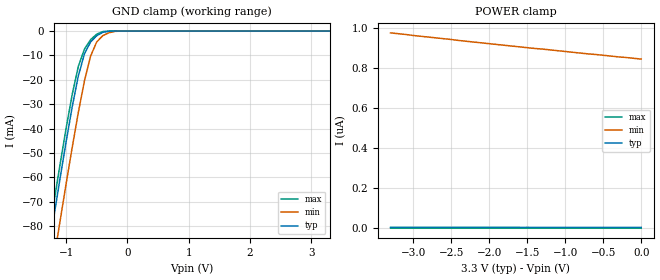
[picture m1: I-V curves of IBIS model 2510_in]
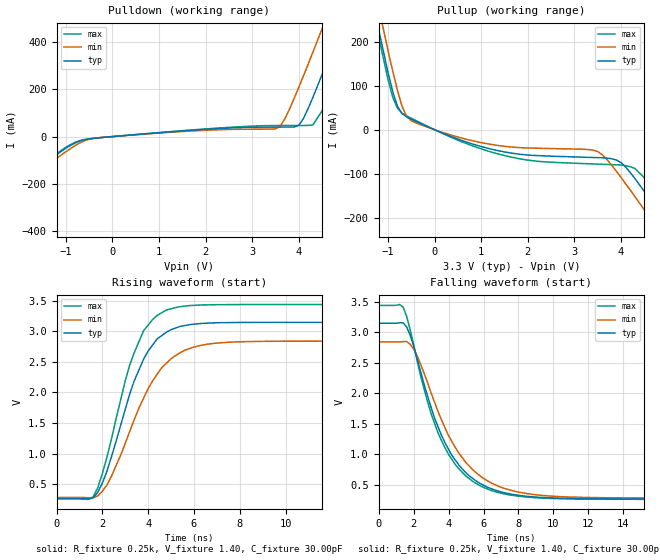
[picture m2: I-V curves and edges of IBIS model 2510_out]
| IBIS file csp2510d.ibs created by s2ibis2 version 1.1
| North Carolina State University Electronics Research Laboratory  1995
[IBIS ver]   2.1
[File name]   csp2510d.ibs
[File Rev]   0.1
[Date]   9/22/99
[Source]   Integrated Device Technology, Inc.
[Notes]   1.Temperatures: typ=25C, min=100C, max=0C 2.Cemos8.5 3vv
   process. 3.RRmp rates based on 50 ohm load.
[Disclaimer] Integrated Device Technology, Inc. ("IDT") hereby grants the
   user of this IBIS model a non-exclusive, nontransferable
   license to use this IBIS model under the following terms. The
   user is granted this license only to use the IBIS model and is
   not granted rights to sell, copy (except as needed to run the
   IBIS model), rent, lease or sub-license the IBIS model in
   whole or in part, or in modified form to anyone. The User may
   modify the IBIS model to suit its specific applications, but
   rights to derivative works and such modifications shall belong
   to IDT. This IBIS model is provided on an AS IS" basis and IDT
   makes absolutely no warranty with respect to the information
   contained herein. IDT DISCLAIMS AND CUSTOMER WAIVES ALL
   WARRANTIES, EXPRESS AND IMPLIED, INCLUDING WARRANTIES OF
   MERCHANTABILITY AND FITNESS FOR A PARTICULAR PURPOSE. THE
   ENTIRE RISK AS TO QUALITY AND PERFORMANCE IS WITH THE USER
   ACCORDINGLY, IN NO EVENT SHALL IDT BE LIABLE FOR ANY DIRECT OR
   INDIRECT DAMAGES, WHETHER IN CONTRACT OR TORT, INCLUDING ANY
   LOST PROFITS OR OTHER INCIDENTAL, CONSEQUENTIAL, EXEMPLARY, OR
   PUNITIVE DAMAGES ARISING OUT OF THE USE OR APPLICATION OF THE
   IBIS model. Further, IDT reserves the right to make changes
   without notice to any product herein to improve reliability,
   function, or design. IDT does not convey any license under
   patent rights or any other intellectual property rights,
   including those of third parties. IDT is not obligated to
   provide maintenance or support for the licensed IBIS model.
[Copyright]   Copyright 1998, Integrated Device Technology, Inc. all rights
   reserved
|   Component IDTCSP2510D
[Component]   IDTCSP2510D
[Manufacturer]   Integrated Device Technology
[Package]
| variable   typ   min   max
R_pkg   10.00m   9.00m   10.50m
L_pkg   0.80nH   82.30pH   8.45nH
C_pkg   0.26pF   0.21pF   0.34pF
[Pin]  signal_name   model_name   R_pin   L_pin   C_pin
1   AGND   GND
2   VDD   POWER
3   Y0   2510_out
13   FBIN   2510_in
| Models and submodels in the file (2): 2510_in (Input), 2510_out (Output)
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| dout dout   dummy_model
|   Model 2510_in
[Model]   2510_in
Model_type   Input
Polarity   Non-Inverting
Vinl =  0.800V
Vinh =  2.200V
Vmeas =  1.500V
C_comp   3.00pF   NA   NA
[Temperature Range]   25.00   100.00   0.000
[Voltage Range]   3.30V   3.00V   3.60V
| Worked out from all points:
|   GND clamp passes 1 mA (typ) near -0.44 V on its own axis
[GND_clamp]
| voltage   I(typ)   I(min)   I(max)
-3.3V     -422mA     -438mA     -416mA
-1.3V     -92.09mA   -110mA     -86.28mA
-1.2V     -76.23mA   -93.85mA   -70.44mA
-1.1V     -60.64mA   -78.15mA   -54.91mA
-900mV    -31.06mA   -47.68mA   -25.93mA
-800mV    -18.37mA   -33.35mA   -14.47mA
-700mV    -9.311mA   -20.38mA   -7.37mA
-600mV    -4.469mA   -10.27mA   -3.514mA
-500mV    -1.887mA   -4.422mA   -1.262mA
-400mV    -508uA     -1.869mA   -183uA
-200mV    -2.072uA   -113uA     -319nA
3.3V      3.982nA    857nA      334pA
[POWER_clamp]
| voltage   I(typ)   I(min)   I(max)
-3.3V     4.913nA    977nA      435pA
-3.1V     4.851nA    969nA      428pA
-3V       4.82nA     964nA      425pA
-2.5V     4.669nA    944nA      410pA
-2.4V     4.639nA    939nA      407pA
-1.4V     4.353nA    899nA      378pA
-1.3V     4.325nA    896nA      376pA
-700mV    4.163nA    872nA      360pA
-600mV    4.137nA    869nA      357pA
-300mV    4.059nA    857nA      349pA
-200mV    4.033nA    854nA      347pA
0V        3.982nA    846nA      342pA
|   Model 2510_out
[Model]   2510_out
Model_type   Output
Polarity   Non-Inverting
Vmeas =  1.500V
C_comp   3.00pF   NA   NA
[Temperature Range]   25.00   100.00   0.000
[Voltage Range]   3.30V   3.00V   3.60V
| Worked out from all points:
|   slope of the pulldown table from 0 to 0.495 V, typ, clamps not added: 60 ohm
|   slope of the pullup table from 0 to 0.495 V, typ, clamps not added: 23.6 ohm
|   rising waveform, R_fixture 0.25k, V_fixture 1.40, C_fixture 30.00pF: 20-80 % time 1.53ns typ, 1.86ns min, 1.4ns max; typ from 0.269 V to 3.15 V
|   falling waveform, R_fixture 0.25k, V_fixture 1.40, C_fixture 30.00pF: 20-80 % time 2.35ns typ, 2.63ns min, 2.24ns max; typ from 3.15 V to 0.269 V
[Pulldown]
| voltage   I(typ)   I(min)   I(max)
-3.3V     -388mA     -405mA     -383mA
-1.5V     -118mA     -135mA     -113mA
-600mV    -13.12mA   -17.48mA   -12.67mA
3.5V      40.03mA    32.79mA    46.54mA
3.7V      40.13mA    75.27mA    46.73mA
4V        47.63mA    209mA      46.9mA
4.3V      165mA      356mA      49.18mA
4.5V      263mA      456mA      109mA
4.9V      464mA      659mA      302mA
5.1V      566mA      762mA      403mA
5.3V      668mA      864mA      504mA
6.6V      1.34A      1.536A     1.174A
[Pullup]
| voltage   I(typ)   I(min)   I(max)
-3.3V     1.299A     1.349A     1.283A
-1.5V     374mA      426mA      357mA
-1V       130mA      180mA      114mA
-800mV    53.78mA    90.57mA    49.52mA
-500mV    24.02mA    20.4mA     26.1mA
1.5V      -50.4mA    -37.59mA   -58.71mA
3.5V      -63.35mA   -49.6mA    -78.08mA
4V        -74.59mA   -108mA     -80.16mA
4.3V      -111mA     -152mA     -88.19mA
4.9V      -200mA     -242mA     -166mA
5.3V      -261mA     -302mA     -226mA
6.6V      -461mA     -501mA     -426mA
[Ramp]
| variable   typ   min   max
dV/dt_r   1.28/0.71n   1.03/0.93n   1.46/0.65n
dV/dt_f   0.87/0.47n   0.73/0.71n   0.97/0.38n
R_load = 50.00
[Rising Waveform]
R_fixture = 0.25k
V_fixture = 1.40
C_fixture = 30.00pF
R_dut = 10.00m
L_dut = 0.80nH
C_dut = 0.26pF
| time   V(typ)   V(min)   V(max)
0s        269mV      286mV      264mV
1.6ns     278mV      283mV      296mV
2.2ns     712mV      489mV      942mV
3ns       1.724V     1.169V     2.189V
3.4ns     2.196V     1.563V     2.654V
3.8ns     2.542V     1.904V     3.006V
4.8ns     2.985V     2.478V     3.347V
6ns       3.116V     2.741V     3.422V
7.6ns     3.141V     2.822V     3.435V
19.8ns    3.145V     2.838V     3.436V
[Falling Waveform]
R_fixture = 0.25k
V_fixture = 1.40
C_fixture = 30.00pF
R_dut = 10.00m
L_dut = 0.80nH
C_dut = 0.26pF
| time   V(typ)   V(min)   V(max)
0s        3.145V     2.838V     3.436V
1.4ns     3.151V     2.844V     3.408V
1.8ns     2.949V     2.801V     3.04V
2.2ns     2.564V     2.613V     2.533V
3.4ns     1.449V     1.698V     1.348V
4.2ns     978mV      1.204V     913mV
5.6ns     559mV      693mV      520mV
7ns       387mV      461mV      364mV
9ns       301mV      338mV      290mV
19.8ns    269mV      286mV      264mV
